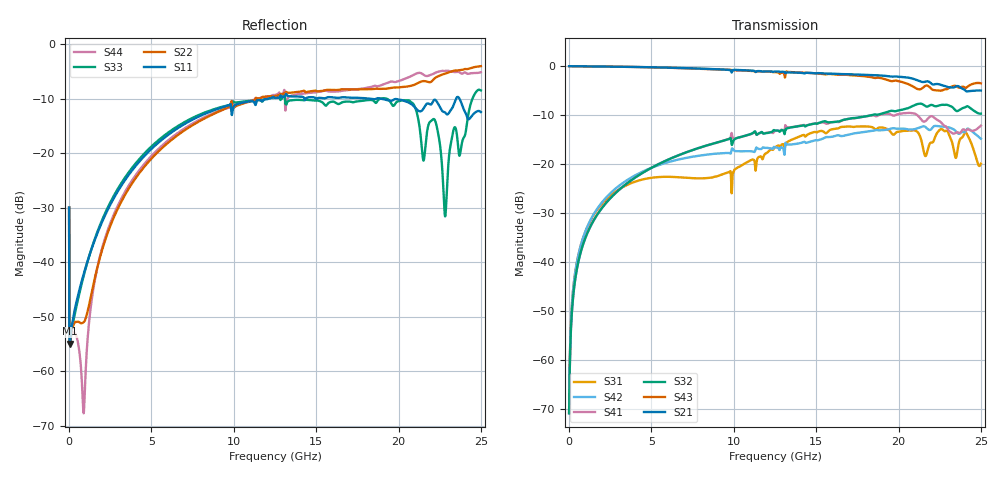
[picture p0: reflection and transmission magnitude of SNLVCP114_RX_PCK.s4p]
! Touchstone Ver. 1.0
! Mon Jun 18 15:05:57 2012
! Number of ports is 4
# Hz	S	MA	R	50.000000
! SCATTERING PARAMETERS  :
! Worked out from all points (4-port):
!   2501 points, 1 MHz to 25 GHz, reference 50 ohm
!   strongest paths, dB at 1 MHz, 6.251 GHz, 12.5 GHz, 18.75 GHz, 25 GHz:
!     S21: 0.0, -0.3, -1.1, -1.9, -5.0
!     S43: 0.0, -0.4, -1.2, -2.3, -3.5
!     S32: -70.9, -18.8, -13.2, -9.9, -9.7
!     S41: -70.9, -18.8, -13.3, -10.1, -12.2
!     S42: -70.8, -19.4, -16.6, -13.1, -14.8
!     S31: -70.8, -22.6, -16.6, -12.7, -19.9
!   lowest |S11| = -54.9 dB at 41 MHz (marker M1), VSWR 1.00, Z = 50.2 - j0.0282 ohm
!   |S11| at or under -10 dB: start of sweep to 12.07 GHz; 18.98 GHz to 23.49 GHz (4.508 GHz wide, 21.2 % of centre); 23.71 GHz to end of sweep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
1000000  0.03179 -85.3  0.9979 1.8  0.0002873 5.5  0.0002843 -174.6
         0.9979 1.8  0.03179 -85.3  0.0002843 -174.6  0.0002874 5.5
         0.0002873 5.5  0.0002843 -174.6  0.0318 -85.4  0.9979 1.8
         0.0002843 -174.6  0.0002874 5.5  0.9979 1.8  0.03179 -85.4
4.1e7  0.001793 -9.0  0.9982 -0.5  0.0009566 65.3  0.0008328 -116.6
       0.9982 -0.5  0.001776 -8.8  0.0008328 -116.6  0.0009584 65.9
       0.0009566 65.3  0.0008328 -116.6  0.001815 -13.6  0.9982 -0.5
       0.0008328 -116.6  0.0009584 65.9  0.9982 -0.5  0.001796 -13.4
8.81e8  0.007744 8.3  0.9944 -10.8  0.01818 72.1  0.0157 -102.5
        0.9944 -10.8  0.002817 74.6  0.0157 -102.5  0.01834 83.2
        0.01818 72.1  0.0157 -102.5  0.007475 -16.0  0.9944 -10.9
        0.0157 -102.5  0.01834 83.2  0.9944 -10.9  0.0004106 -83.0
3.951e9  0.07373 -54.3  0.9806 -48.0  0.06552 13.8  0.07158 -139.7
         0.9806 -48.0  0.05663 134.6  0.07156 -139.6  0.07564 67.1
         0.06552 13.8  0.07156 -139.6  0.07781 -64.0  0.9801 -48.4
         0.07158 -139.7  0.07564 67.1  0.9801 -48.4  0.0602 145.6
1.4511e10  0.3266 122.2  0.8537 -173.1  0.2011 81.0  0.2508 79.4
           0.8537 -173.1  0.3681 57.3  0.2501 81.6  0.1667 44.9
           0.2011 81.0  0.2501 81.6  0.3089 113.8  0.8521 -174.8
           0.2508 79.4  0.1667 44.9  0.8521 -174.8  0.3575 59.4
2.2831e10  0.2372 -67.3  0.627 81.7  0.2164 145.0  0.2439 -47.2
           0.627 81.7  0.538 45.3  0.4021 -45.1  0.2391 14.5
           0.2164 145.0  0.4021 -45.1  0.02634 118.7  0.5797 97.2
           0.2439 -47.2  0.2391 14.5  0.5797 97.2  0.5695 32.1
2.5001e10  0.2391 -100.2  0.5633 59.6  0.1008 95.4  0.2464 -46.7
           0.5633 59.6  0.6309 36.2  0.3268 -79.9  0.1811 0.8
           0.1008 95.4  0.3268 -79.9  0.3781 -57.8  0.6661 70.7
           0.2464 -46.7  0.1811 0.8  0.6661 70.7  0.555 26.6
